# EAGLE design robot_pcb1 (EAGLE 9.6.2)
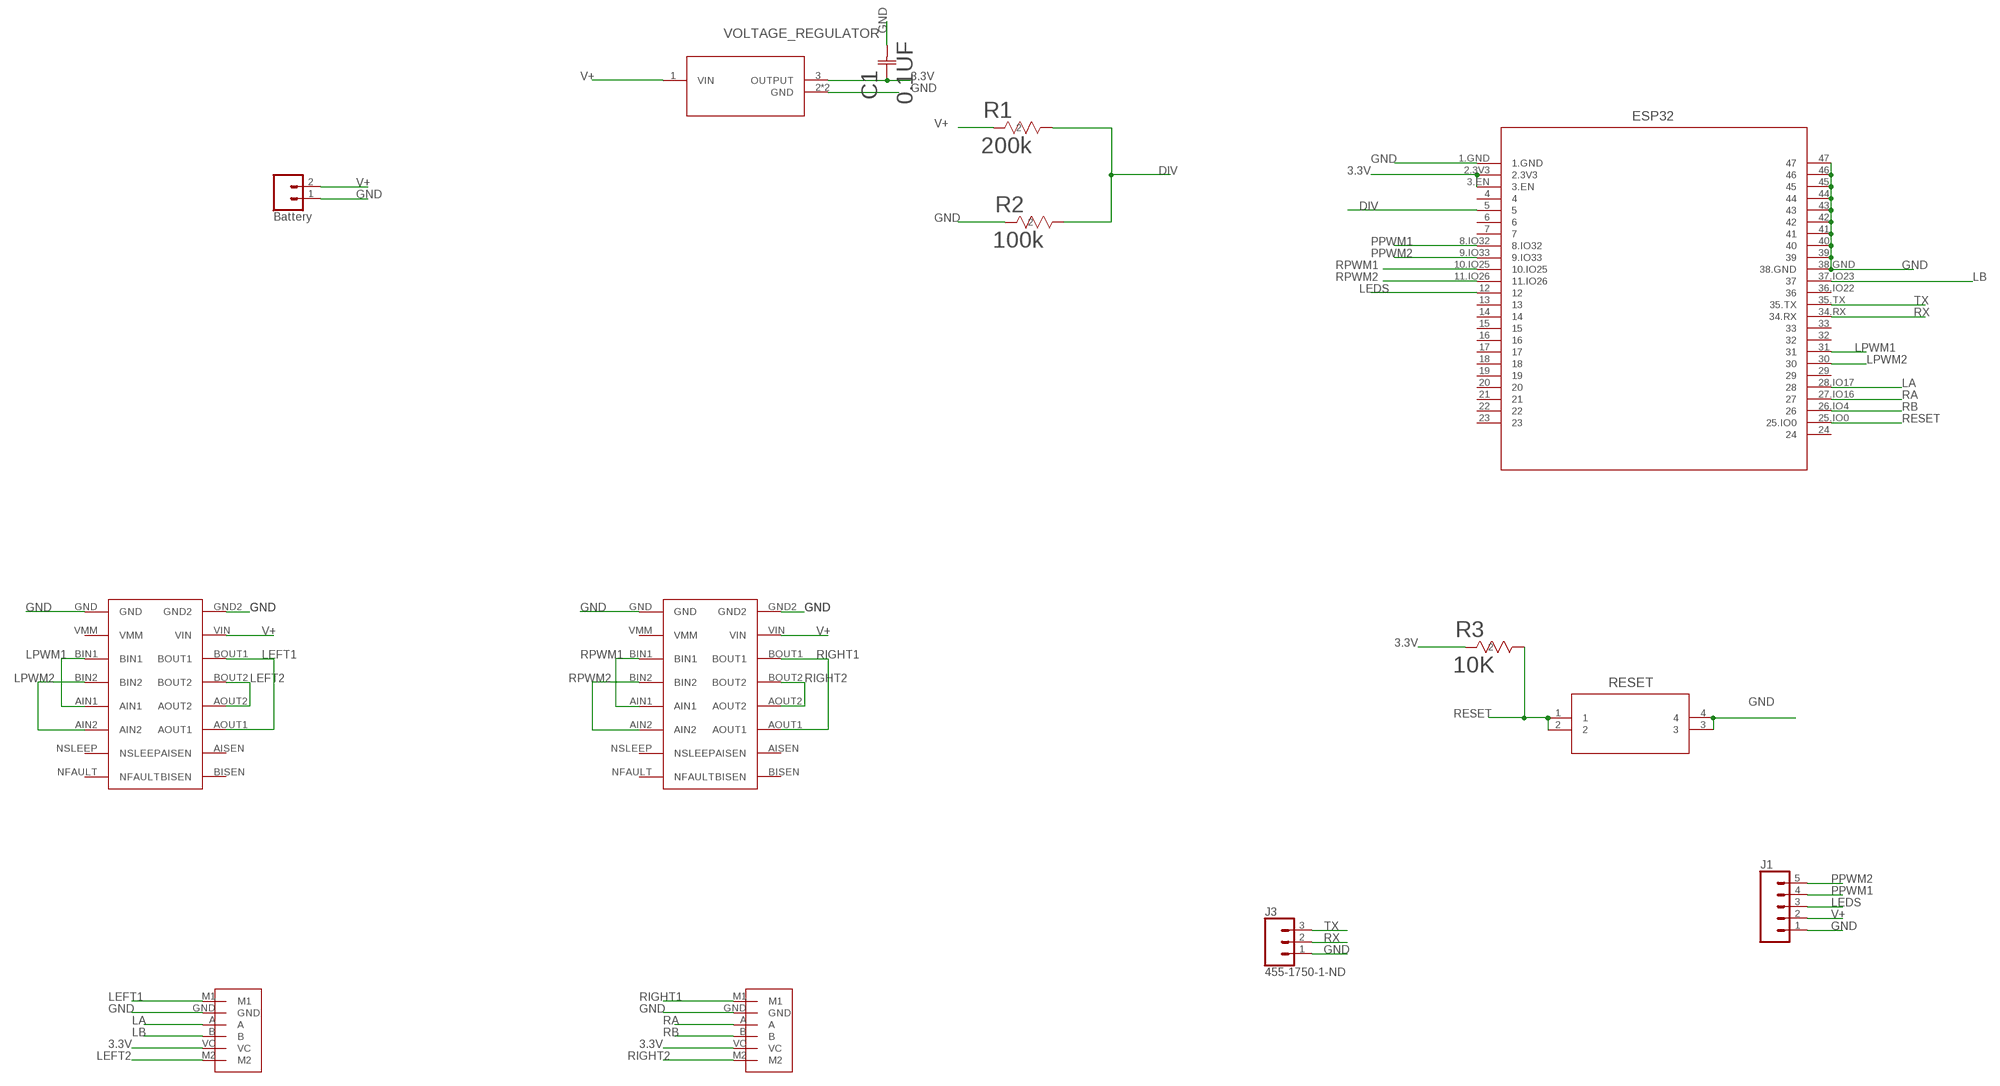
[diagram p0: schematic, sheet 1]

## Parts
C1  0.1UF  CAP0603  [CAP0603]
ESP32  ESP32  [ESP32]
J1  CONN_05  [1X05]
J2  Battery  CONN_02  [CONN_02]
J3  455-1750-1-ND  CONN_03  [1X03]
R1  200k  RES0603  [RES0603]
R2  100k  RES0603  [RES0603]
R3  10K  RES0603  [RES0603]
RESET  PUSH_BUTTONSMT_FS-M  [PUSH_BUTTON]
U$1  MOTOR_CONNECTOR  [MOTOR_CONNECTOR]
U$2  MOTOR_CONNECTOR  [MOTOR_CONNECTOR]
U$5  DRV8833_BREAKOUT  [DRV8833_BREAKOUT]
U$6  DRV8833_BREAKOUT  [DRV8833_BREAKOUT]
VOLTAGE_REGULATOR  VOLTAGE_REGULATORSOT-223_ST_LIT-L  [VOLTAGE_REGULATOR]

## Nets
3.3V: C1.1 ESP32.2.3V3 ESP32.3.EN R3.2 U$1.VC U$2.VC VOLTAGE_REGULATOR.3(OUTPUT)
DIV: ESP32.5 R1.1 R2.1
GND: C1.2 ESP32.1.GND ESP32.38.GND ESP32.39 ESP32.40 ESP32.41 ESP32.42 ESP32.43 ESP32.44 ESP32.45 ESP32.46 ESP32.47 J1.1 J2.1 J3.1 R2.2 RESET.3 RESET.4 U$1.GND U$2.GND U$5.GND U$5.GND2 U$6.GND U$6.GND2 VOLTAGE_REGULATOR.2(GND) VOLTAGE_REGULATOR.4(GND)
LA: ESP32.28.IO17 U$1.A
LB: ESP32.37.IO23 U$1.B
LEDS: ESP32.12 J1.3
LEFT1: U$1.M1 U$5.AOUT1 U$5.BOUT1
LEFT2: U$1.M2 U$5.AOUT2 U$5.BOUT2
LPWM1: ESP32.31 U$5.AIN1 U$5.BIN1
LPWM2: ESP32.30 U$5.AIN2 U$5.BIN2
PPWM1: ESP32.8.IO32 J1.4
PPWM2: ESP32.9.IO33 J1.5
RA: ESP32.27.IO16 U$2.A
RB: ESP32.26.IO4 U$2.B
RESET: ESP32.25.IO0 R3.1 RESET.1 RESET.2
RIGHT1: U$2.M1 U$6.AOUT1 U$6.BOUT1
RIGHT2: U$2.M2 U$6.AOUT2 U$6.BOUT2
RPWM1: ESP32.10.IO25 U$6.AIN1 U$6.BIN1
RPWM2: ESP32.11.IO26 U$6.AIN2 U$6.BIN2
RX: ESP32.34.RX J3.2
TX: ESP32.35.TX J3.3
V+: J1.2 J2.2 R1.2 U$5.VIN U$6.VIN VOLTAGE_REGULATOR.1(VIN)
Unconnected: ESP32.4 ESP32.6 ESP32.7 ESP32.13 ESP32.14 ESP32.15 ESP32.16 ESP32.17 ESP32.18 ESP32.19 ESP32.20 ESP32.21 ESP32.22 ESP32.23 ESP32.24 ESP32.29 ESP32.32 ESP32.33 ESP32.36.IO22 U$5.AISEN U$5.BISEN U$5.NFAULT U$5.NSLEEP U$5.VMM U$6.AISEN U$6.BISEN U$6.NFAULT U$6.NSLEEP U$6.VMM

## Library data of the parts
C1 = maciver_robot_lib:CAP0603; BUILT_BY: EMA_UL_Team; COPYRIGHT: Copyright (C) 2018 Accelerated Designs. All rights reserved; MANUFACTURER_PART_NUMBER: 0603YC105KAT2A; SOURCELIBRARY: AVX_2015-1-12; VENDOR: AVX Corporation
ESP32 = maciver_robot_lib:ESP32; BUILT_BY: EMA_Kyle; COPYRIGHT: Copyright (C) 2018 Accelerated Designs. All rights reserved; DATASHEET: https://www.espressif.com/sites/default/files/documentation/esp32-wroom-32_datasheet_en.pdf; MANUFACTURER_PART_NUMBER: ESP32-WROOM-32 (8MB); SOURCELIBRARY: Add_to_database_2020-12-29; VENDOR: Espressif Systems
J1 = maciver_robot_lib:CONN_05: Multi connection point. Often used as Generic Header-pin footprint for 0.1 inch spaced/style header connections On any of the 0.1 inch spaced packages, you can populate with these: Break Away Headers - Straight (PRT-00116) Break Away Male Headers - Right Angle (PRT-00553) Female Headers (PRT-00115)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
J2 = maciver_robot_lib:CONN_02: Multi connection point. Often used as Generic Header-pin footprint for 0.1 inch spaced/style header connections
J3 = SparkFun-Connectors:CONN_03: Multi connection point. Often used as Generic Header-pin footprint for 0.1 inch spaced/style header connections On any of the 0.1 inch spaced packages, you can populate with these: Break Away Headers - Straight (PRT-00116) Break Away Male Headers - Right Angle (PRT-00553) Female Headers (PRT-00115)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; PROD_ID: XXX-00000
R1-R3 = maciver_robot_lib:RES0603; BUILT_BY: EMA_UL_Team; MANUFACTURER_PART_NUMBER: ERJ-3GEYJ103V; SOURCELIBRARY: Panasonic_2010-01-01_Res5; VENDOR: Panasonic
RESET = maciver_robot_lib:PUSH_BUTTON; BUILT_BY: EMA_Matt; COPYRIGHT: Copyright (C) 2018 Accelerated Designs. All rights reserved; MANUFACTURER_PART_NUMBER: PTS526 SK15 SMTR2 LFS; SOURCELIBRARY: C&K_2019-11-15; VENDOR: C&K
U$1 U$2 = maciver_robot_lib:MOTOR_CONNECTOR
U$5 U$6 = maciver_robot_lib:DRV8833_BREAKOUT
VOLTAGE_REGULATOR = maciver_robot_lib:VOLTAGE_REGULATOR; COPYRIGHT: Copyright (C) 2022 Ultra Librarian. All rights reserved.; DIGI-KEY_PART_NUMBER_1: LT1129IST-3.3#TRPBFCT-ND; DIGI-KEY_PART_NUMBER_2: LT1129IST-3.3#TRPBFDKR-ND; DIGI-KEY_PART_NUMBER_3: LT1129IST-3.3#TRPBFTR-ND; MANUFACTURER_PART_NUMBER: LT1129IST-3.3#TRPBF; MFR_NAME: Analog Devices / Linear Technology

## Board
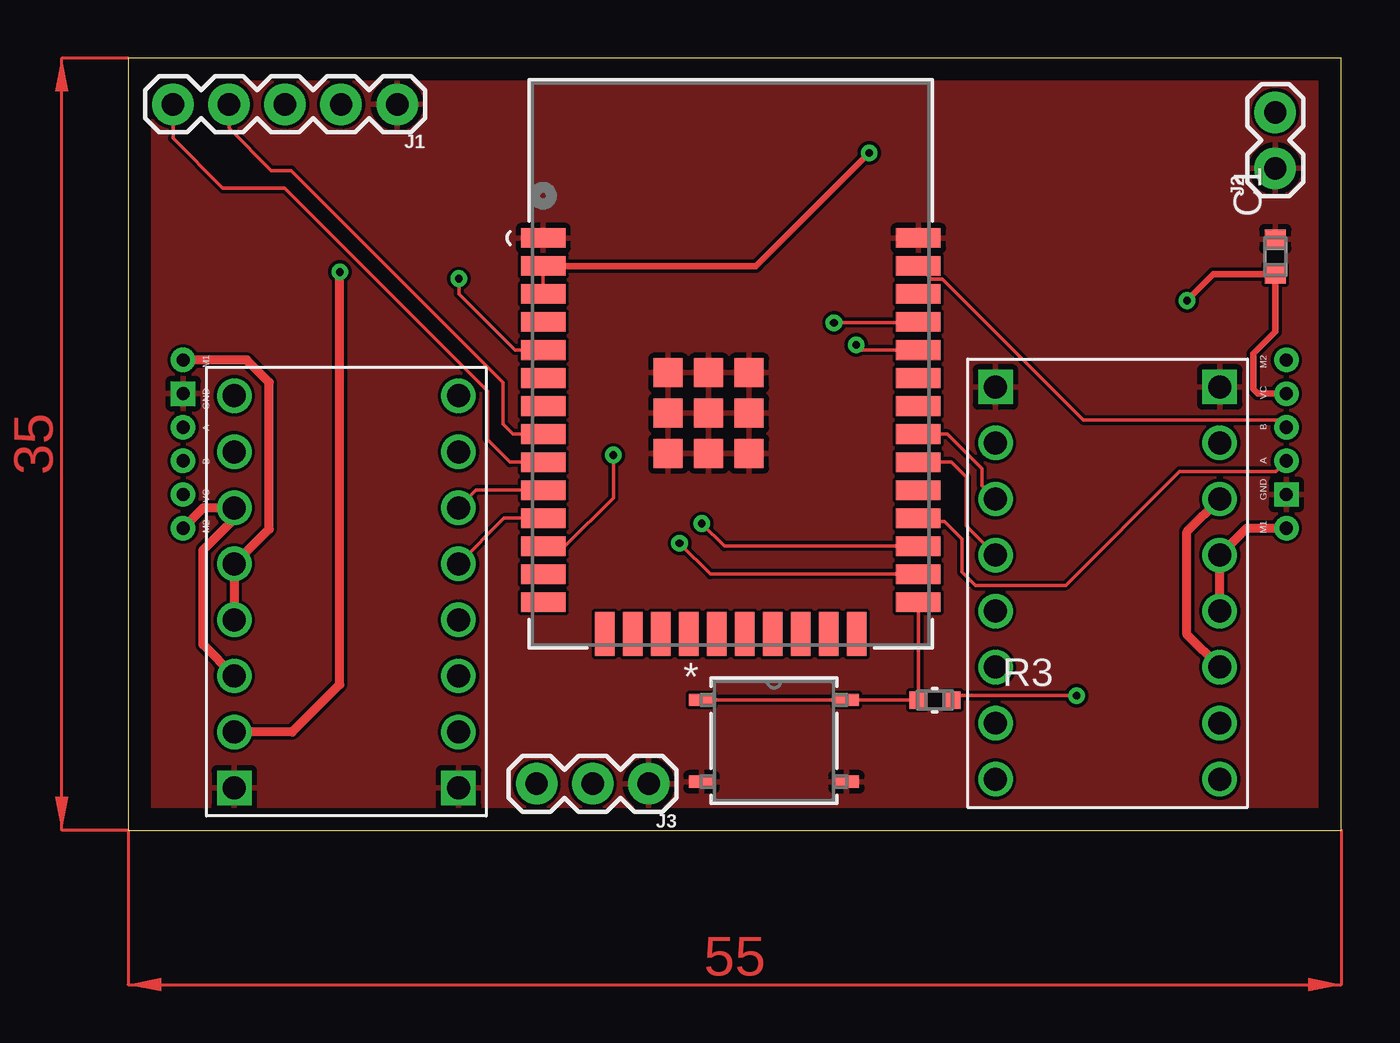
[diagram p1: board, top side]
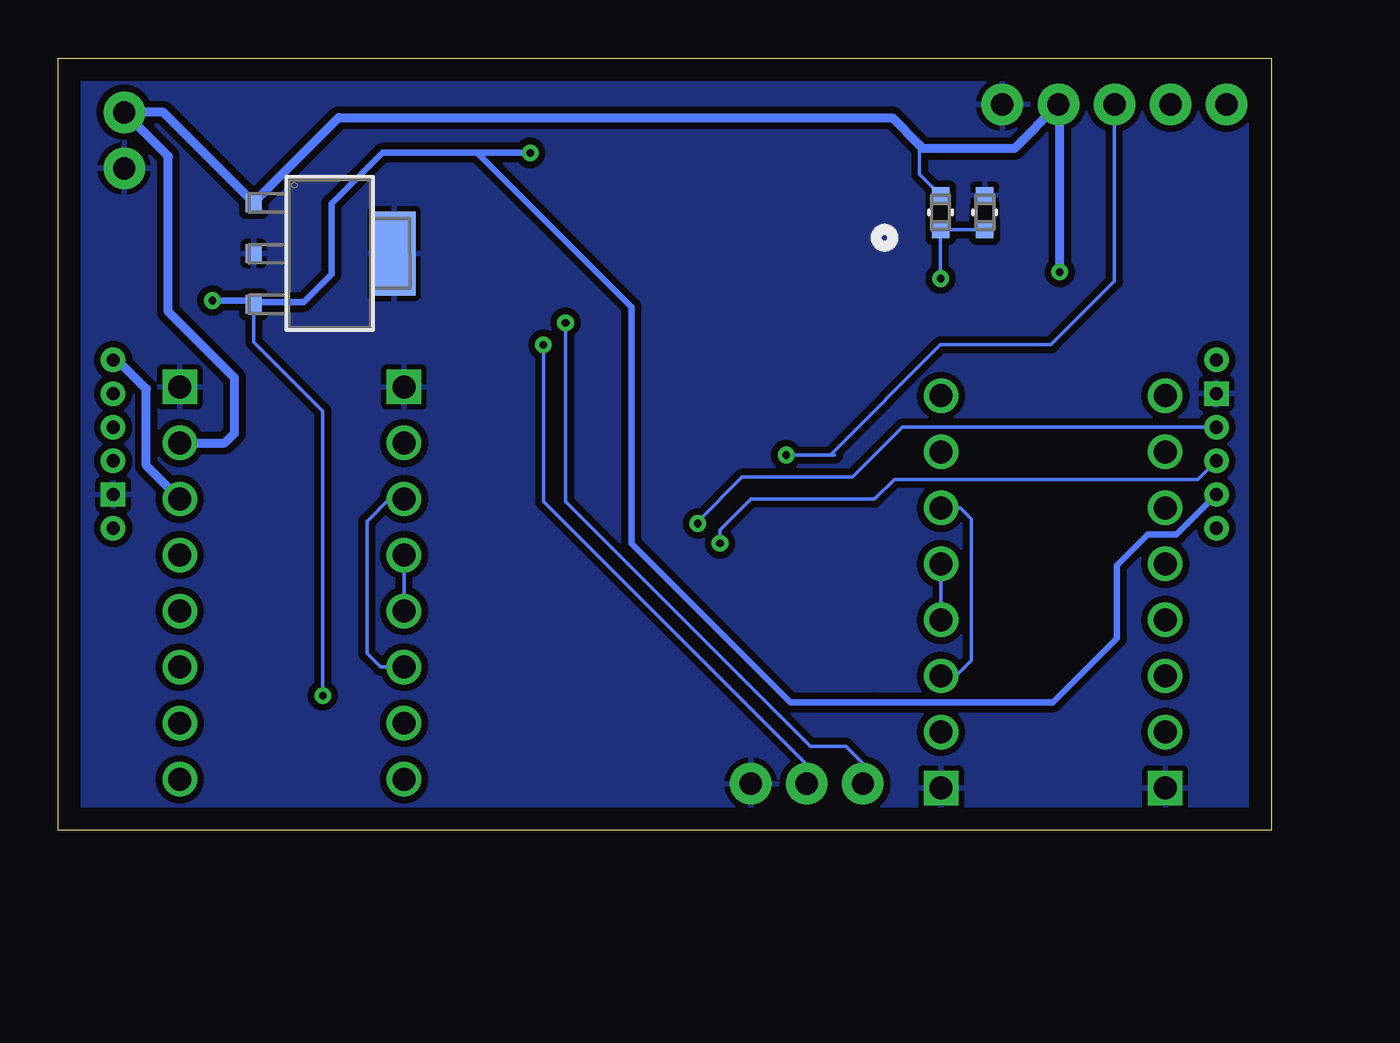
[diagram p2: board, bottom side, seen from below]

Size 55 x 35 mm. Coordinates in mm from the lower left corner, seen from the top.
Outline: 0,0 55,0 55,35 0,35 0,0
Copper layers (1*16): Top 0.035mm / dielectric 1.5mm / Bottom 0.035mm
Design rules "default": minimum track width 6mil, minimum drill 0.35mm, track to track 6mil, track to pad 6mil, pad to pad 6mil, via to via 6mil, smd to smd 6mil, copper to edge 40mil, drill to drill 6mil, minimum pad ring 10mil, minimum via ring 8mil, stop-mask expansion 4mil, vias tented up to drill 0mil, thermal gap 10mil

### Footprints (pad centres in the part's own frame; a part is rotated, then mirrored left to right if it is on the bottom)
CAP0603 = smd 0.864 x 0.965: 1 -0.8,0; 2 0.8,0
ESP32 = smd 2.007 x 0.889: 1.GND -8.5,5.704; 2.3V3 -8.5,4.434; 3.EN -8.5,3.164; 4 -8.5,1.894; 5 -8.5,0.624; 6 -8.5,-0.646; 7 -8.5,-1.916; 8.IO32 -8.5,-3.186; 9.IO33 -8.5,-4.456; 10.IO25 -8.5,-5.726; 11.IO26 -8.5,-6.996; 12 -8.5,-8.266; 13 -8.5,-9.536; 14 -8.5,-10.806; 25.IO0 8.5,-10.806; 26.IO4 8.5,-9.536; 27.IO16 8.5,-8.266; 28.IO17 8.5,-6.996; 29 8.5,-5.726; 30 8.5,-4.456; 31 8.5,-3.186; 32 8.5,-1.916; 33 8.5,-0.646; 34.RX 8.5,0.624; 35.TX 8.5,1.894; 36.IO22 8.5,3.164; 37.IO23 8.5,4.434; 38.GND 8.5,5.704 | smd 0.889 x 2.007: 15 -5.715,-12.248; 16 -4.445,-12.248; 17 -3.175,-12.248; 18 -1.905,-12.248; 19 -0.635,-12.248; 20 0.635,-12.248; 21 1.905,-12.248; 22 3.175,-12.248; 23 4.445,-12.248; 24 5.715,-12.248 | smd 1.321 x 1.321: 39 -2.839,-0.405; 40 -1.004,-0.405; 41 0.831,-0.405; 42 -2.839,-2.24; 43 -1.004,-2.24; 44 0.831,-2.24; 45 -2.839,-4.075; 46 -1.004,-4.075; 47 0.831,-4.075
1X05 = drill 1.016 pad 1.88: 1 0,0; 2 2.54,0; 3 5.08,0; 4 7.62,0; 5 10.16,0
CONN_02 = drill 1.016 pad 1.88: 1 0,0; 2 2.54,0
1X03 = drill 1.016 pad 1.88: 1 0,0; 2 2.54,0; 3 5.08,0
RES0603 = smd 0.756 x 0.8: 1 -0.778,0; 2 0.778,0
PUSH_BUTTON = smd 1.156 x 0.559: 1 -3.283,1.854; 2 3.283,1.854; 3 -3.283,-1.854; 4 3.283,-1.854
MOTOR_CONNECTOR = drill 0.6: A -0.762,0; B 0.762,0; M1 3.81,0; M2 -3.81,0; VC 2.286,0 | drill 0.6 square: GND -2.286,0
DRV8833_BREAKOUT = drill 1.04: AIN1 -5.08,-3.81; AIN2 -5.08,-1.27; AISEN 5.08,-6.35; AOUT1 5.08,-3.81; AOUT2 5.08,-1.27; BIN1 -5.08,3.81; BIN2 -5.08,1.27; BISEN 5.08,-8.89; BOUT1 5.08,3.81; BOUT2 5.08,1.27; NFAULT -5.08,-8.89; NSLEEP -5.08,-6.35; VIN 5.08,6.35; VMM -5.08,6.35 | drill 1.04 square: GND -5.08,8.89; GND2 5.08,8.89
VOLTAGE_REGULATOR = smd 0.838 x 0.711: 1 -2.299,-3.442; 2 0,-3.442; 3 2.299,-3.442 | smd 3.81 x 1.93: 4 0,2.921

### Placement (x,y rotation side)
C1  52,26 90 top
ESP32  27.32,21.14 0 top
J1  12.2,32.9 180 top
J2  52,30 90 top
J3  23.6,2.1 180 top
R1  15,28 90 bottom
R2  13,28 90 bottom
R3  36.57,5.9 0 top
RESET  29.28,4.05 0 top
U$1  52.5,17.5 90 top
U$2  2.5,17.5 270 top
U$5  44.4,11.2 0 top
U$6  9.9,10.8 180 top
VOLTAGE_REGULATOR  42.69,26.14 270 bottom

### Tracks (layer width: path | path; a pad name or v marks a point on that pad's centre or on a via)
3.3V  (via drill 0.35)
  Top 0.152: ESP32.3.EN ESP32.2.3V3 | 37.55,6.1 v43,6.1
  Top 0.305: v33.6,30.7 28.47,25.57 ESP32.2.3V3 | R3.2 37.55,6.1 | v48,24 49.2,25.2 C1.1 52,22.6 51,21.6 51,20 51.21,19.79 U$1.VC
  Bottom 0.152: VOLTAGE_REGULATOR.3 46.13,22.13 43,19 v43,6.1
  Bottom 0.305: 46.03,23.94 43.86,23.94 42.6,25.2 42.6,28.4 40.3,30.7 36,30.7 | VOLTAGE_REGULATOR.3 46.29,24 v48,24 | U$2.VC 4.31,13.4 5.6,13.4 7,12 7,8.7 9.9,5.8 18,5.8 21.8,5.8 29,13 29,23.7 36,30.7 | v33.6,30.7 36,30.7
  Bottom 0.406: VOLTAGE_REGULATOR.3 46.03,23.94
DIV  (via drill 0.35)
  Top 0.152: ESP32.5 17.54,21.76 15,24.3 v15,25
  Bottom 0.152: v15,25 R1.1 R2.1
GND
  pour Top: 0,35 0,0 55,0 55,35
  pour Top (isolate 0.305): 0,35 55,35 55,0 0,0
  pour Bottom (isolate 0.305): 0,0 0,35 55,35 55,0
LA
  Top 0.152: ESP32.28.IO17 35.96,14 37,14 37.8,13.2 37.8,11.7 38.4,11.1 42.5,11.1 47.66,16.26 52.02,16.26 U$1.A
LB
  Top 0.152: ESP32.37.IO23 36.42,24.98 36.92,24.98 43.3,18.6 52.16,18.6 U$1.B
LEDS  (via drill 0.35)
  Top 0.152: ESP32.12 19.82,12.87 22,15.05 v22,17
  Bottom 0.152: v22,17 20,17 | 20,17 19.8,17 | 20,17 15,22 10,22 7.12,24.88 J1.3
LEFT1
  Top 0.406: U$5.AOUT1 48,8.87 48,13.53 U$5.BOUT1
  Bottom 0.406: U$5.BOUT1 51,16.53 51,20 52.31,21.31 U$1.M1
LEFT2
  Top 0.406: U$5.AOUT2 U$5.BOUT2 50.7,13.69 U$1.M2
LPWM1
  Top 0.152: U$5.BIN1 38.7,15.63 38.7,16.4 37.15,17.95 ESP32.31
  Bottom 0.152: U$5.AIN1 40.39,7.39 41,8 41,14 39.99,15.01 U$5.BIN1
LPWM2
  Top 0.152: U$5.BIN2 38,13.79 38,16 37.32,16.68 ESP32.30
  Bottom 0.152: U$5.AIN2 U$5.BIN2
PPWM1
  Top 0.152: ESP32.8.IO32 17.45,17.95 17,18.4 17,20.3 7.4,29.9 6.5,29.9 4.58,31.82 J1.4
PPWM2
  Top 0.152: ESP32.9.IO33 17.32,16.68 16.3,17.7 16.3,19.9 7.1,29.1 4.3,29.1 2.04,31.36 J1.5
RA  (via drill 0.35)
  Top 0.152: ESP32.27.IO16 27.03,12.87 v26,13.9
  Bottom 0.152: v26,13.9 26,14 24,16 19,16 16.74,18.26 U$2.A
RB  (via drill 0.35)
  Top 0.152: ESP32.26.IO4 26.4,11.6 v25,13
  Bottom 0.152: U$2.B 3.34,15.9 17.1,15.9 18,15 23.6,15 25,13.6 v25,13
RESET
  Top 0.152: RESET.2 | RESET.2 RESET.1 | ESP32.25.IO0 35.82,5.93 R3.1 RESET.2
RIGHT1
  Top 0.406: U$2.M1 3.42,14.61 U$6.AOUT1 4.82,14.11 3.4,12.69 3.4,8.41 U$6.BOUT1
RIGHT2
  Top 0.406: U$6.BOUT2 U$6.AOUT2 6.4,13.65 6.4,20.3 5.39,21.31 U$2.M2
RPWM1
  Top 0.152: ESP32.10.IO25 15.78,15.41 U$6.AIN1
  Bottom 0.152: U$6.BIN1 14.31,6.99 13.6,7.7 13.6,14.1 14.11,14.61 U$6.AIN1
RPWM2
  Top 0.152: ESP32.11.IO26 17.05,14.14 U$6.AIN2
  Bottom 0.152: U$6.BIN2 U$6.AIN2
RX  (via drill 0.35)
  Top 0.152: ESP32.34.RX 33.24,21.76 v33,22
  Bottom 0.152: v33,22 33,14.9 21.06,2.96 J3.2
TX  (via drill 0.35)
  Top 0.152: ESP32.35.TX 35.79,23 v32,23
  Bottom 0.152: v32,23 32,14.9 20.9,3.8 19.3,3.8 18.52,3.02 J3.3
V+  (via drill 0.35)
  Top 0.406: U$6.VIN 7.45,4.45 9.6,6.6 v9.6,25.3
  Bottom 0.152: 15.95,31.05 15.95,29.73 R1.2
  Bottom 0.406: 42.27,32.3 42.28,32.28 | 42.28,32.28 VOLTAGE_REGULATOR.1 50.23,32.54 J2.2 50,30.54 50,23.5 47,20.5 47,18 47.45,17.55 U$5.VIN | 42.28,32.28 17.18,32.28 15.95,31.05 15.8,30.9 11.66,30.9 J1.2 9.6,32.84 v9.6,25.3
(copper drawn outside any net)
  shapes: Top area x2

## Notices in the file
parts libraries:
SparkFun-Connectors: Licensing: Creative Commons ShareAlike 4.0 International - https://creativecommons.org/licenses/by-sa/4.0
